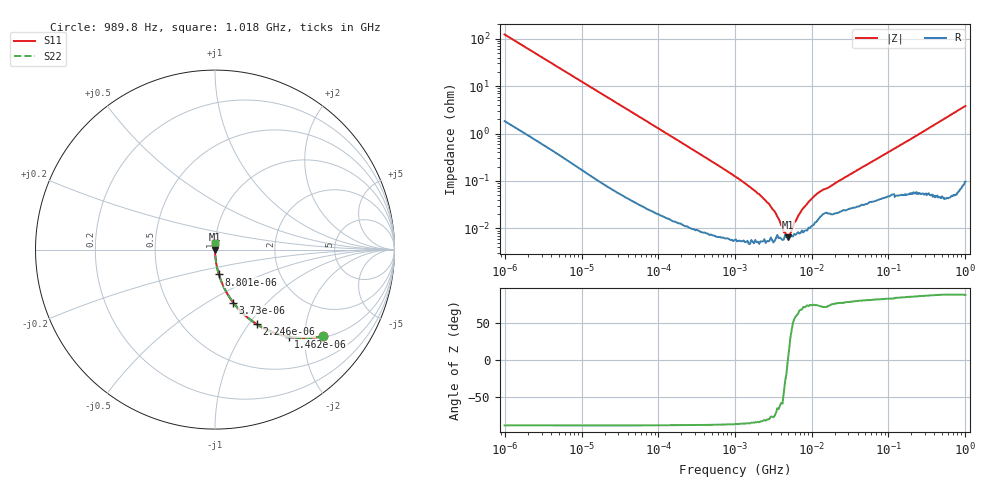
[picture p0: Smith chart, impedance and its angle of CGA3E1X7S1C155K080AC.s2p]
! S-Parameter Data Generated by TDK Corporation
! Copyright(C) 2024 TDK Corporation.
! All Rights Reserved.
! TDK P/N: CGA3E1X7S1C155K080AC (Multilayer Ceramic Chip Capacitor)
! Property: C=1.5uF
! Size(LxWxT): 1.6x0.8x0.8mm
! Model Type: s2p (Touchstone File Format Version 1.0)
! Frequency: DC=Yes Start=0.000989846MHz Stop=1017.91MHz 409points Log-sweep
! Model Generated on May 28, 2024
! Terms and conditions regarding TDK Simulation Models:
! 1)This simulation model is being provided solely for informational
!  purposes. Please refer to the specifications of the products in
!  terms of detailed characteristics of such products.
! 2)In no event shall TDK Corporation of any of its subsidiaries be
!  liable for any loss or damage arising, directly or indirectly,
!  from any information contained in this simulation model, including,
!  but not limited to loss or damages arising from any inaccuracies,
!  omissions or errors in connection with such information.
! 3)Any and all copyrights on this simulation model are owned by
!  TDK Corporation.  Duplication or redistribution of this simulation
!  model without prior written permission from TDK Corporation
!  is prohibited.
! 4)This simulation model is subject to any modification or change
!  without any prior notice.
! 5)Neither TDK Corporation nor any of its subsidiaries shall make any
!  warranty, express or implied, including but not limited to the
!  correctness, implied warranties of merchantability and fitness for
!  a particular purpose with respect to this simulation models.
! 6)The use of this simulation model shall be deemed to have consented
!  to the terms and conditions hereof.
! Port Assignments:
!  1 ---| |--- 2
! Applicable Conditions:
!  Temperature = 25 degC
!  DC Bias Voltage = 0 V
!  Small Signal Operation
# Hz S MA R 50
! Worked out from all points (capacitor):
!   408 points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, 989.8 Hz to 1.018 GHz, reference 50 ohm
!   read as one part in series: C = 1.31 uF near 1.07 kHz
!   lowest |Z| = 6.52 mohm at 4.894 MHz (marker M1)
!   series resonance near 4.91 MHz, so ESL is about 800 pH
!   S11 on the Smith chart (normalised r, x): 989.8 Hz: 1.04, -2.45; 1.462 kHz: 1.02, -1.67; 2.246 kHz: 1.02, -1.09; 3.73 kHz: 1.01, -0.66; 8.801 kHz: 1.00, -0.28; 1.018 GHz: 1.00, +0.08
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989.846  0.7695 -38.8  0.6273 50.3  0.6273 50.3  0.7695 -38.8
1462.25  0.6354 -49.7  0.7627 39.4  0.7627 39.4  0.6354 -49.7
2246.06  0.4753 -60.8  0.8727 28.4  0.8727 28.4  0.4753 -60.8
3730.02  0.312 -71.0  0.9455 18.2  0.9455 18.2  0.312 -71.0
8800.53  0.1402 -81.1  0.9882 8.1  0.9882 8.1  0.1402 -81.1
10287  0.1206 -82.3  0.9911 6.9  0.9911 6.9  0.1206 -82.3
26241  0.0483 -86.5  0.9982 2.8  0.9982 2.8  0.0483 -86.5
102818  0.01252 -88.4  0.9997 0.7  0.9997 0.7  0.01252 -88.4
1027650  0.00122 -87.2  0.9999 0.1  0.9999 0.1  0.00122 -87.2
1518090  0.0007788 -86.5  1 0.0  1 0.0  0.0007788 -86.5
2242600  0.0004678 -83.5  0.9999 0.0  0.9999 0.0  0.0004678 -83.5
3064190  0.0002599 -77.5  0.9999 0.0  0.9999 0.0  0.0002599 -77.5
4186770  0.0001125 -59.5  0.9999 0.0  0.9999 0.0  0.0001125 -59.5
4353360  8.252e-05 -44.8  0.9999 0.0  0.9999 0.0  8.252e-05 -44.8
4893960  6.517e-05 -1.3  0.9999 0.0  0.9999 0.0  6.517e-05 -1.3
5291160  7.747e-05 29.7  0.9999 -0.0  0.9999 -0.0  7.747e-05 29.7
5720600  0.000106 50.5  0.9999 -0.0  0.9999 -0.0  0.000106 50.5
7229600  0.000221 68.4  0.9999 -0.0  0.9999 -0.0  0.000221 68.4
1.02712e7  0.0004347 74.7  0.9999 -0.0  0.9999 -0.0  0.0004347 74.7
1.29806e7  0.0006024 73.1  0.9998 -0.0  0.9998 -0.0  0.0006024 73.1
1.0266e8  0.00413 83.2  0.9995 -0.2  0.9995 -0.2  0.00413 83.2
1.01791e9  0.03807 86.4  0.9983 -2.2  0.9983 -2.2  0.03807 86.4
